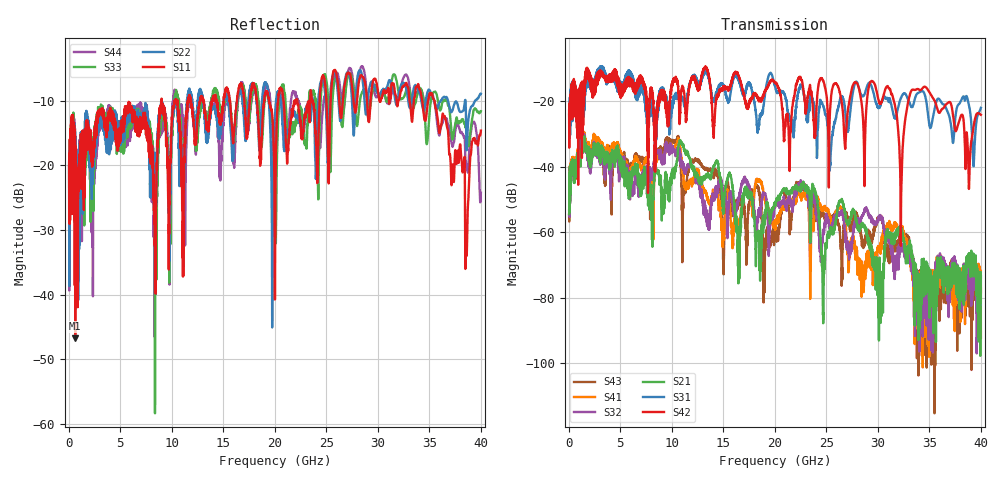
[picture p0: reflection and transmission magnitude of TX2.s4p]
!Agilent Technologies,N5245A,MY49151084,A.09.00.04
!Agilent N5245A: A.09.00.04
!Date: Thursday, January 20, 2011 08:57:56
!Correction: S11(Full 4 Port(1,2,3,4))
!S12(Full 4 Port(1,2,3,4))
!S13(Full 4 Port(1,2,3,4))
!S14(Full 4 Port(1,2,3,4))
!S21(Full 4 Port(1,2,3,4))
!S22(Full 4 Port(1,2,3,4))
!S23(Full 4 Port(1,2,3,4))
!S24(Full 4 Port(1,2,3,4))
!S31(Full 4 Port(1,2,3,4))
!S32(Full 4 Port(1,2,3,4))
!S33(Full 4 Port(1,2,3,4))
!S34(Full 4 Port(1,2,3,4))
!S41(Full 4 Port(1,2,3,4))
!S42(Full 4 Port(1,2,3,4))
!S43(Full 4 Port(1,2,3,4))
!S44(Full 4 Port(1,2,3,4))
!S4P File: Measurements: <S11,S12,S13,S14>,
!<S21,S22,S23,S24>,
!<S31,S32,S33,S34>,
!<S41,S42,S43,S44>:
# Hz S  dB  R 50
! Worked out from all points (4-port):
!   3996 points, 50 MHz to 40 GHz, reference 50 ohm
!   strongest paths, dB at 50 MHz, 10.04 GHz, 20.03 GHz, 30.02 GHz, 40 GHz:
!     S42: -23.0, -14.9, -14.4, -19.1, -24.2
!     S31: -24.1, -20.8, -15.7, -21.8, -22.1
!     S21: -54.5, -42.9, -50.9, -79.2, -73.4
!     S32: -53.5, -35.1, -52.5, -57.0, -77.3
!     S41: -54.4, -34.8, -56.8, -65.8, -78.4
!     S43: -55.2, -33.0, -57.6, -56.3, -92.2
!   lowest |S11| = -46.8 dB at 640 MHz (marker M1), VSWR 1.01, Z = 49.6 - j0.101 ohm
!   |S11| at or under -10 dB: start of sweep to 9.015 GHz; 9.024 GHz to 10.29 GHz (1.27 GHz wide, 13.2 % of centre); 35.49 GHz to end of sweep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
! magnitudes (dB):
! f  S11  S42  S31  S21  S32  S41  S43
! 50 MHz  -20.1  -23.0  -24.1  -54.5  -53.5  -54.4  -55.2
! 640 MHz  -46.8  -22.6  -21.4  -43.4  -43.1  -42.3  -43.9
! 10.54 GHz  -9.9  -14.2  -18.2  -37.8  -36.4  -32.7  -31.6
! 18.99 GHz  -10.0  -17.3  -19.8  -57.2  -48.2  -48.7  -77.0
! 22.37 GHz  -11.5  -12.9  -16.1  -46.7  -45.6  -47.7  -45.2
! 32.25 GHz  -8.4  -52.8  -19.1  -59.0  -66.0  -59.6  -61.0
! 40 GHz  -14.6  -24.2  -22.1  -73.4  -77.3  -78.4  -92.2
